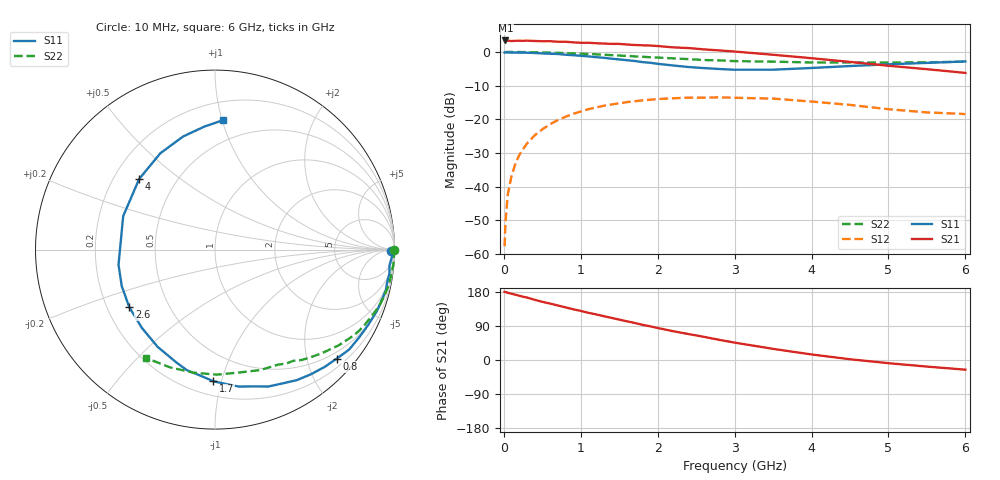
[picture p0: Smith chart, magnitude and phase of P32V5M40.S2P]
! SIEMENS Small Signal Semiconductors
! BFP181
! Si NPN RF Bipolar Junction Transistor in SOT143
! VCE = 2.5 V  IC = 0.4 mA
! Common Emitter S-Parameters:  March  1996
# GHz  S  MA  R  50
!  f  S11  S21  S12  S22
! GHz  MAG  ANG  MAG  ANG  MAG  ANG  MAG  ANG
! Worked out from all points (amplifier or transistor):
!   36 points, 10 MHz to 6 GHz, reference 50 ohm
!   highest |S21| = 3.4 dB at 20 MHz (marker M1)
!   |S21| within 3 dB of that: start of sweep to 2.823 GHz
!   unconditionally stable (mu >= 1): 3.845 GHz to end of sweep
!   at 250 MHz: K = 0.08, MSG = 16.1 dB, |S12| = -28.9 dB
!   at 1.4 GHz: K = 0.43, MSG = 9.0 dB, |S12| = -15.6 dB
!   at 6 GHz: K = 1.52, MAG = 1.9 dB, |S12| = -18.5 dB
!   S11 on the Smith chart (normalised r, x): 10 MHz: 83, -48; 800 MHz: 0.36, -2.57; 1.7 GHz: 0.30, -0.94; 2.6 GHz: 0.29, -0.28; 4 GHz: 0.31, +0.36; 6 GHz: 0.33, +1.01
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0.01  0.9821 -0.6  1.467 179.8  0.0013 87.7  0.9999 -0.2
0.02  0.9858 -1.2  1.481 179.6  0.0028 84.1  0.9919 -0.5
0.05  0.9864 -2.4  1.472 177.5  0.0075 91.7  0.9976 -1.3
0.1  0.976 -5.2  1.451 174.9  0.0144 87.4  0.9978 -2.6
0.15  0.981 -7.9  1.464 172.3  0.0218 84.5  0.9972 -3.9
0.2  0.9762 -10.5  1.466 169.6  0.0293 82.5  0.9966 -5.2
0.3  0.9729 -15.8  1.471 164.9  0.0435 79.0  0.9939 -7.7
0.4  0.9646 -20.8  1.456 158.9  0.0576 74.8  0.9894 -10.3
0.6  0.9402 -31.4  1.444 148.9  0.0842 67.0  0.9771 -15.3
0.8  0.9103 -41.9  1.418 139.1  0.1085 59.7  0.961 -20.2
1.1  0.8584 -57.9  1.369 124.5  0.1411 49.0  0.9318 -27.1
1.5  0.7746 -80.1  1.317 106.6  0.1725 36.0  0.8826 -35.6
1.7  0.7336 -90.7  1.269 97.8  0.1849 30.1  0.8584 -39.5
1.9  0.6903 -103.0  1.246 89.0  0.1949 24.3  0.8351 -43.1
2.2  0.6292 -120.5  1.169 76.0  0.2049 16.5  0.8028 -48.3
2.6  0.5754 -146.1  1.092 61.2  0.2091 7.0  0.758 -54.8
3  0.544 -171.1  1.014 45.9  0.2084 -2.5  0.7306 -61.3
3.5  0.5444 160.0  0.908 29.4  0.2026 -11.9  0.717 -69.4
4  0.5775 137.0  0.807 14.6  0.1831 -19.4  0.6979 -78.8
4.5  0.6173 119.5  0.711 2.0  0.1633 -25.0  0.6968 -89.2
5.5  0.6877 95.0  0.554 -17.4  0.1264 -23.1  0.7025 -111.0
6  0.7228 86.4  0.488 -25.5  0.1194 -18.4  0.7151 -122.3
